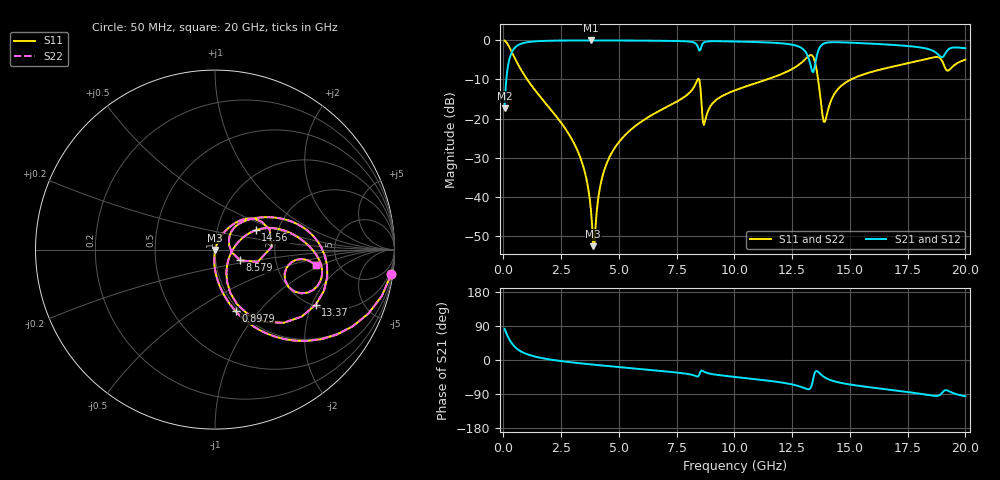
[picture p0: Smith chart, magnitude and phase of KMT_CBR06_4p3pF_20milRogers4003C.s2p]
! Data measured by Modelithics Inc. support@modelithics.com 813-866-6335
! KEMET CBR0603 4.3pF, Pad Width= 0.851mm, Pad Length= 0.64mm, Pad Gap= 0.62mm, 20mil Rogers 4003C substrate Data, January 2022
# hz S ma R 50
! 2 Port Network Data from SP1.SP block
! freq  magS11  angS11  magS21  angS21  magS12  angS12  magS22  angS22
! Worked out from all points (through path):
!   401 points, 50 MHz to 20 GHz, reference 50 ohm
!   highest |S21| = -0.02 dB at 3.791 GHz (marker M1); lowest = -17.4 dB at 50 MHz (marker M2)
!   group delay of S21, straight-line fit = 15.7 ps
!   lowest |S11| = -52.7 dB at 3.89 GHz (marker M3), VSWR 1.00, Z = 50.2 - j0.162 ohm
!   |S11| at or under -10 dB: 1.028 GHz to 8.411 GHz (7.383 GHz wide, 156 % of centre); 8.48 GHz to 11.41 GHz (2.929 GHz wide, 29.5 % of centre); 13.62 GHz to 15.05 GHz (1.425 GHz wide, 9.94 % of centre)
!   |S22| runs from -52.7 to -0.1 dB; largest |S21 - S12| = 0
!   S11 on the Smith chart (normalised r, x): 50 MHz: 1, -14; 897.9 MHz: 0.96, -0.76; 8.579 GHz: 1.32, -0.16; 13.37 GHz: 2.06, -2.14; 14.56 GHz: 1.54, +0.36; 20 GHz: 3.38, -0.87
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5e7  0.9908 -7.9  0.1349 82.1  0.1349 82.1  0.9908 -7.9
3.4925e8  0.7216 -44.9  0.6916 45.1  0.6916 45.1  0.7216 -44.9
8.97875e8  0.3617 -71.5  0.9312 18.3  0.9312 18.3  0.3617 -71.5
3.391625e9  0.02794 -95.4  0.9976 -9.2  0.9976 -9.2  0.02794 -95.4
3.790625e9  0.006592 -84.4  0.9979 -11.7  0.9979 -11.7  0.006592 -84.4
3.890375e9  0.002323 -44.0  0.9979 -12.3  0.9979 -12.3  0.002323 -44.0
4.2395e9  0.01591 68.2  0.9977 -14.3  0.9977 -14.3  0.01591 68.2
4.688375e9  0.03636 69.6  0.997 -16.9  0.997 -16.9  0.03636 69.6
6.73325e9  0.1246 60.2  0.9889 -28.4  0.9889 -28.4  0.1246 60.2
8.379125e9  0.3035 30.6  0.8723 -43.3  0.8723 -43.3  0.3035 30.6
8.578625e9  0.1527 -23.2  0.8474 -27.7  0.8474 -27.7  0.1527 -23.2
8.72825e9  0.09233 33.0  0.9575 -32.2  0.9575 -32.2  0.09233 33.0
1.0025e10  0.2295 44.0  0.9677 -44.7  0.9677 -44.7  0.2295 44.0
1.271825e10  0.4714 18.2  0.8486 -67.7  0.8486 -67.7  0.4714 18.2
1.306738e10  0.5742 4.5  0.7208 -75.1  0.7208 -75.1  0.5742 4.5
1.336662e10  0.6399 -28.7  0.402 -62.4  0.402 -62.4  0.6399 -28.7
1.366588e10  0.2549 -70.6  0.7838 -33.7  0.7838 -33.7  0.2549 -70.6
1.391525e10  0.09072 -13.0  0.9223 -46.1  0.9223 -46.1  0.09072 -13.0
1.456362e10  0.2521 25.4  0.946 -59.8  0.946 -59.8  0.2521 25.4
1.670825e10  0.4511 10.2  0.8814 -78.4  0.8814 -78.4  0.4511 10.2
1.895262e10  0.5711 -24.8  0.6106 -89.3  0.6106 -89.3  0.5711 -24.8
2e10  0.5671 -8.8  0.7936 -95.8  0.7936 -95.8  0.5671 -8.8
